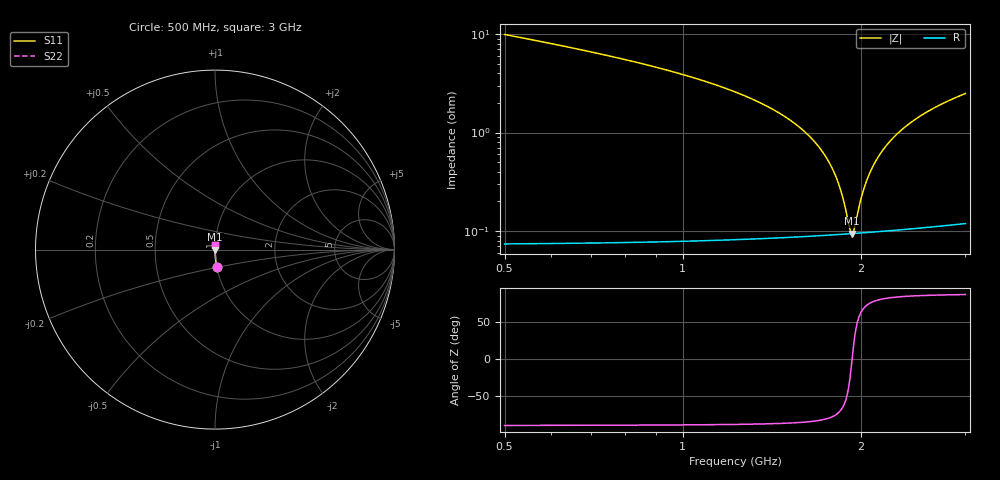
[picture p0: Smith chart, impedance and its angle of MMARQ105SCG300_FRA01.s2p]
! MMARQ105SCG300_FRA01  S-PARAMETER MODEL  ( General Type )
! Model Generated by TAIYO YUDEN Corporation (http://www.ty-top.com)
! Version 1.0
! TAIYO YUDEN Control No. 200326
! Copyright(c) 2020 TAIYO YUDEN CO.,LTD. All Rights Reserved.
! Product Description (link to TY-COMPAS)
! https://ds.yuden.co.jp/TYCOMPAS/or/detail?pn=MMARQ105SCG300JFRA01&u=M
! Products Name : Multilayer Ceramic Capacitors
! Characteristics :
!  Capacitance : 30 pF , Rated Voltage : 250V , TCC : CG / C0G
!  Case Size : 1.0 x 0.5 / 0.039 x 0.02 [mm/inch] , Thickness : 0.5 / 0.02 [mm/inch]
!  (Conditions: Temperature = 25 degC , DC Bias Current/Voltage = 0A / 0V)
! External Node Assignments :
!  1  o---| |---o  2
! GND o---------o GND
! Frequency Range : 500MHz  -  3GHz  [ 401 STEP ]
# MHz S RI R 50
! Freq[MHz].  S11 Real  S11 Imag  S21 Real  S21 Imag  S12 Real  S12 Imag  S22 Real  S22 Imag
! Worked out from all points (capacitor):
!   401 points, 500 MHz to 3 GHz, reference 50 ohm
!   read as one part in series: C = 30 pF near 512.5 MHz
!   lowest |Z| = 94.3 mohm at 1.931 GHz (marker M1)
!   series resonance near 1.931 GHz, so ESL is about 230 pH
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500  0.0104 -0.0978  0.9896 0.0978  0.9896 0.0978  0.0104 -0.0978
918.75  0.00276 -0.0445  0.9972 0.0445  0.9972 0.0445  0.00276 -0.0445
1337.5  0.00126 -0.0206  0.9987 0.0206  0.9987 0.0206  0.00126 -0.0206
1475  0.00108 -0.0149  0.9989 0.0149  0.9989 0.0149  0.00108 -0.0149
1587.5  0.000992 -0.0108  0.999 0.0108  0.999 0.0108  0.000992 -0.0108
1675  0.000953 -0.00781  0.999 0.00781  0.999 0.00781  0.000953 -0.00781
1750  0.000935 -0.00539  0.9991 0.00539  0.9991 0.00539  0.000935 -0.00539
1793.75  0.000931 -0.00404  0.9991 0.00404  0.9991 0.00404  0.000931 -0.00404
1831.25  0.00093 -0.0029  0.9991 0.0029  0.9991 0.0029  0.00093 -0.0029
1868.75  0.000933 -0.00179  0.9991 0.00179  0.9991 0.00179  0.000933 -0.00179
1912.5  0.000939 -0.000526  0.9991 0.000526  0.9991 0.000526  0.000939 -0.000526
1931.25  0.000942 7.25e-06  0.9991 -7.25e-06  0.9991 -7.25e-06  0.000942 7.25e-06
1950  0.000946 0.000535  0.9991 -0.000535  0.9991 -0.000535  0.000946 0.000535
2000  0.00096 0.00192  0.999 -0.00192  0.999 -0.00192  0.00096 0.00192
2043.75  0.000975 0.0031  0.999 -0.0031  0.999 -0.0031  0.000975 0.0031
2100  0.000999 0.00459  0.999 -0.00459  0.999 -0.00459  0.000999 0.00459
2168.75  0.00103 0.00636  0.999 -0.00636  0.999 -0.00636  0.00103 0.00636
2250  0.00108 0.00838  0.9989 -0.00838  0.9989 -0.00838  0.00108 0.00838
2343.75  0.00115 0.0106  0.9989 -0.0106  0.9989 -0.0106  0.00115 0.0106
2587.5  0.00135 0.0162  0.9986 -0.0162  0.9986 -0.0162  0.00135 0.0162
2781.25  0.00155 0.0203  0.9984 -0.0203  0.9984 -0.0203  0.00155 0.0203
3000  0.00181 0.0248  0.9982 -0.0248  0.9982 -0.0248  0.00181 0.0248
